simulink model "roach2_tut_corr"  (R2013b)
settings: Solver=VariableStepDiscrete  SolverMode=SingleTasking  StartTime=0.0  StopTime=100  RelTol=1e-3
undefined symbols (not defined in the file): add_latency, addr_width, Bit, bitfield, BitWidth, bram_latency, burst_size, casper_library_scopes, conv_latency, data_width, DelayLen, fan_latency, FFTSize, FFTStage, getfield, increment, led, Location, Lower, mult_latency, mux_latency, n_bits, n_bits_data, n_inputs, n_streams, n_taps, neg_latency, negate_latency, nsamples, pfb_size, pulse_len, reset_period, ROACH, ROACH2, snapshot, sx475t, sync_period, sync_period_bits, Upper, UseCounter, Width
libraries: xbsIndex_r4 x24444, casper_library_misc x73, xbsReplacements_r4 x34, casper_library_delays x14, xps_library x7
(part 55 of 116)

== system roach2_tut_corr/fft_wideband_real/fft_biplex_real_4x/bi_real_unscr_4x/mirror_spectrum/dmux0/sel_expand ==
  bus_in : Inport
  reinterpret{1..4} (4 alike) : xbsIndex_r4/Reinterpret  force_arith_type=on  arith_type=Unsigned  force_bin_pt=on  bin_pt=0  block_type=reinterpret
  slice1 : xbsIndex_r4/Slice  nbits=1  boolean_output=off  mode=Upper Bit Location + Width  bit1=-3  base1=MSB of Input  bit0=0  base0=LSB of Input  dbl_ovrd=off  block_type=slice
  slice2 : xbsIndex_r4/Slice  nbits=1  boolean_output=off  mode=Upper Bit Location + Width  bit1=-2  base1=MSB of Input  bit0=0  base0=LSB of Input  dbl_ovrd=off  block_type=slice
  slice3 : xbsIndex_r4/Slice  nbits=1  boolean_output=off  mode=Upper Bit Location + Width  bit1=-1  base1=MSB of Input  bit0=0  base0=LSB of Input  dbl_ovrd=off  block_type=slice
  slice4 : xbsIndex_r4/Slice  nbits=1  boolean_output=off  mode=Upper Bit Location + Width  bit1=0  base1=MSB of Input  bit0=0  base0=LSB of Input  dbl_ovrd=off  block_type=slice
  msb_out4 : Outport
  out3 : Outport  Port=2
  out2 : Outport  Port=3
  lsb_out1 : Outport  Port=4
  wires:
  bus_in/1 -> slice4/1, slice3/1, slice2/1, slice1/1
  slice4/1 -> reinterpret4/1
  reinterpret4/1 -> msb_out4/1
  slice3/1 -> reinterpret3/1
  reinterpret3/1 -> out3/1
  slice2/1 -> reinterpret2/1
  reinterpret2/1 -> out2/1
  slice1/1 -> reinterpret1/1
  reinterpret1/1 -> lsb_out1/1

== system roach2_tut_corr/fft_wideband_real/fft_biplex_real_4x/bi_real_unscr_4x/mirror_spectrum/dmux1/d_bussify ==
  in1 : Inport
  in2 : Inport  Port=2
  in3 : Inport  Port=3
  in4 : Inport  Port=4
  concatenate : xbsIndex_r4/Concat  num_inputs=4  dbl_ovrd=off  block_type=concat
  reinterpret{1..4} (4 alike) : xbsIndex_r4/Reinterpret  force_arith_type=on  arith_type=Unsigned  force_bin_pt=on  bin_pt=0  block_type=reinterpret
  bus_out : Outport
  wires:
  concatenate/1 -> bus_out/1
  in1/1 -> reinterpret1/1
  reinterpret1/1 -> concatenate/1
  in2/1 -> reinterpret2/1
  reinterpret2/1 -> concatenate/2
  in3/1 -> reinterpret3/1
  reinterpret3/1 -> concatenate/3
  in4/1 -> reinterpret4/1
  reinterpret4/1 -> concatenate/4

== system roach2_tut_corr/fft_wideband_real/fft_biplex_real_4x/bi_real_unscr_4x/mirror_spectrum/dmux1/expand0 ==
  bus_in : Inport
  reinterpret{1..4} (4 alike) : xbsIndex_r4/Reinterpret  force_arith_type=on  arith_type=Unsigned  force_bin_pt=on  bin_pt=0  block_type=reinterpret
  slice1 : xbsIndex_r4/Slice  nbits=36  boolean_output=off  mode=Upper Bit Location + Width  bit1=-108  base1=MSB of Input  bit0=0  base0=LSB of Input  dbl_ovrd=off  block_type=slice
  slice2 : xbsIndex_r4/Slice  nbits=36  boolean_output=off  mode=Upper Bit Location + Width  bit1=-72  base1=MSB of Input  bit0=0  base0=LSB of Input  dbl_ovrd=off  block_type=slice
  slice3 : xbsIndex_r4/Slice  nbits=36  boolean_output=off  mode=Upper Bit Location + Width  bit1=-36  base1=MSB of Input  bit0=0  base0=LSB of Input  dbl_ovrd=off  block_type=slice
  slice4 : xbsIndex_r4/Slice  nbits=36  boolean_output=off  mode=Upper Bit Location + Width  bit1=0  base1=MSB of Input  bit0=0  base0=LSB of Input  dbl_ovrd=off  block_type=slice
  msb_out4 : Outport
  out3 : Outport  Port=2
  out2 : Outport  Port=3
  lsb_out1 : Outport  Port=4
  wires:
  bus_in/1 -> slice4/1, slice3/1, slice2/1, slice1/1
  slice4/1 -> reinterpret4/1
  reinterpret4/1 -> msb_out4/1
  slice3/1 -> reinterpret3/1
  reinterpret3/1 -> out3/1
  slice2/1 -> reinterpret2/1
  reinterpret2/1 -> out2/1
  slice1/1 -> reinterpret1/1
  reinterpret1/1 -> lsb_out1/1

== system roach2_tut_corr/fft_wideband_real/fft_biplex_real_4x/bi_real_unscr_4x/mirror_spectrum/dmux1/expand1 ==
  bus_in : Inport
  reinterpret{1..4} (4 alike) : xbsIndex_r4/Reinterpret  force_arith_type=on  arith_type=Unsigned  force_bin_pt=on  bin_pt=0  block_type=reinterpret
  slice1 : xbsIndex_r4/Slice  nbits=36  boolean_output=off  mode=Upper Bit Location + Width  bit1=-108  base1=MSB of Input  bit0=0  base0=LSB of Input  dbl_ovrd=off  block_type=slice
  slice2 : xbsIndex_r4/Slice  nbits=36  boolean_output=off  mode=Upper Bit Location + Width  bit1=-72  base1=MSB of Input  bit0=0  base0=LSB of Input  dbl_ovrd=off  block_type=slice
  slice3 : xbsIndex_r4/Slice  nbits=36  boolean_output=off  mode=Upper Bit Location + Width  bit1=-36  base1=MSB of Input  bit0=0  base0=LSB of Input  dbl_ovrd=off  block_type=slice
  slice4 : xbsIndex_r4/Slice  nbits=36  boolean_output=off  mode=Upper Bit Location + Width  bit1=0  base1=MSB of Input  bit0=0  base0=LSB of Input  dbl_ovrd=off  block_type=slice
  msb_out4 : Outport
  out3 : Outport  Port=2
  out2 : Outport  Port=3
  lsb_out1 : Outport  Port=4
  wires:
  bus_in/1 -> slice4/1, slice3/1, slice2/1, slice1/1
  slice4/1 -> reinterpret4/1
  reinterpret4/1 -> msb_out4/1
  slice3/1 -> reinterpret3/1
  reinterpret3/1 -> out3/1
  slice2/1 -> reinterpret2/1
  reinterpret2/1 -> out2/1
  slice1/1 -> reinterpret1/1
  reinterpret1/1 -> lsb_out1/1

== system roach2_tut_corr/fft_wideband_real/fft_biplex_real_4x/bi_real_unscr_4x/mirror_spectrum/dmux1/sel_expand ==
  bus_in : Inport
  reinterpret{1..4} (4 alike) : xbsIndex_r4/Reinterpret  force_arith_type=on  arith_type=Unsigned  force_bin_pt=on  bin_pt=0  block_type=reinterpret
  slice1 : xbsIndex_r4/Slice  nbits=1  boolean_output=off  mode=Upper Bit Location + Width  bit1=-3  base1=MSB of Input  bit0=0  base0=LSB of Input  dbl_ovrd=off  block_type=slice
  slice2 : xbsIndex_r4/Slice  nbits=1  boolean_output=off  mode=Upper Bit Location + Width  bit1=-2  base1=MSB of Input  bit0=0  base0=LSB of Input  dbl_ovrd=off  block_type=slice
  slice3 : xbsIndex_r4/Slice  nbits=1  boolean_output=off  mode=Upper Bit Location + Width  bit1=-1  base1=MSB of Input  bit0=0  base0=LSB of Input  dbl_ovrd=off  block_type=slice
  slice4 : xbsIndex_r4/Slice  nbits=1  boolean_output=off  mode=Upper Bit Location + Width  bit1=0  base1=MSB of Input  bit0=0  base0=LSB of Input  dbl_ovrd=off  block_type=slice
  msb_out4 : Outport
  out3 : Outport  Port=2
  out2 : Outport  Port=3
  lsb_out1 : Outport  Port=4
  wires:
  bus_in/1 -> slice4/1, slice3/1, slice2/1, slice1/1
  slice4/1 -> reinterpret4/1
  reinterpret4/1 -> msb_out4/1
  slice3/1 -> reinterpret3/1
  reinterpret3/1 -> out3/1
  slice2/1 -> reinterpret2/1
  reinterpret2/1 -> out2/1
  slice1/1 -> reinterpret1/1
  reinterpret1/1 -> lsb_out1/1

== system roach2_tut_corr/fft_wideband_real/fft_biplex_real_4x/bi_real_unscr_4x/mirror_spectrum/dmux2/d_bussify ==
  in1 : Inport
  in2 : Inport  Port=2
  in3 : Inport  Port=3
  in4 : Inport  Port=4
  concatenate : xbsIndex_r4/Concat  num_inputs=4  dbl_ovrd=off  block_type=concat
  reinterpret{1..4} (4 alike) : xbsIndex_r4/Reinterpret  force_arith_type=on  arith_type=Unsigned  force_bin_pt=on  bin_pt=0  block_type=reinterpret
  bus_out : Outport
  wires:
  concatenate/1 -> bus_out/1
  in1/1 -> reinterpret1/1
  reinterpret1/1 -> concatenate/1
  in2/1 -> reinterpret2/1
  reinterpret2/1 -> concatenate/2
  in3/1 -> reinterpret3/1
  reinterpret3/1 -> concatenate/3
  in4/1 -> reinterpret4/1
  reinterpret4/1 -> concatenate/4

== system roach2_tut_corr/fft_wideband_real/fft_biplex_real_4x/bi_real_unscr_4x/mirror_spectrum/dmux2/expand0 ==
  bus_in : Inport
  reinterpret{1..4} (4 alike) : xbsIndex_r4/Reinterpret  force_arith_type=on  arith_type=Unsigned  force_bin_pt=on  bin_pt=0  block_type=reinterpret
  slice1 : xbsIndex_r4/Slice  nbits=36  boolean_output=off  mode=Upper Bit Location + Width  bit1=-108  base1=MSB of Input  bit0=0  base0=LSB of Input  dbl_ovrd=off  block_type=slice
  slice2 : xbsIndex_r4/Slice  nbits=36  boolean_output=off  mode=Upper Bit Location + Width  bit1=-72  base1=MSB of Input  bit0=0  base0=LSB of Input  dbl_ovrd=off  block_type=slice
  slice3 : xbsIndex_r4/Slice  nbits=36  boolean_output=off  mode=Upper Bit Location + Width  bit1=-36  base1=MSB of Input  bit0=0  base0=LSB of Input  dbl_ovrd=off  block_type=slice
  slice4 : xbsIndex_r4/Slice  nbits=36  boolean_output=off  mode=Upper Bit Location + Width  bit1=0  base1=MSB of Input  bit0=0  base0=LSB of Input  dbl_ovrd=off  block_type=slice
  msb_out4 : Outport
  out3 : Outport  Port=2
  out2 : Outport  Port=3
  lsb_out1 : Outport  Port=4
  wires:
  bus_in/1 -> slice4/1, slice3/1, slice2/1, slice1/1
  slice4/1 -> reinterpret4/1
  reinterpret4/1 -> msb_out4/1
  slice3/1 -> reinterpret3/1
  reinterpret3/1 -> out3/1
  slice2/1 -> reinterpret2/1
  reinterpret2/1 -> out2/1
  slice1/1 -> reinterpret1/1
  reinterpret1/1 -> lsb_out1/1

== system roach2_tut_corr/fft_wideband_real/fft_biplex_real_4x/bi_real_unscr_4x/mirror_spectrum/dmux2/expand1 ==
  bus_in : Inport
  reinterpret{1..4} (4 alike) : xbsIndex_r4/Reinterpret  force_arith_type=on  arith_type=Unsigned  force_bin_pt=on  bin_pt=0  block_type=reinterpret
  slice1 : xbsIndex_r4/Slice  nbits=36  boolean_output=off  mode=Upper Bit Location + Width  bit1=-108  base1=MSB of Input  bit0=0  base0=LSB of Input  dbl_ovrd=off  block_type=slice
  slice2 : xbsIndex_r4/Slice  nbits=36  boolean_output=off  mode=Upper Bit Location + Width  bit1=-72  base1=MSB of Input  bit0=0  base0=LSB of Input  dbl_ovrd=off  block_type=slice
  slice3 : xbsIndex_r4/Slice  nbits=36  boolean_output=off  mode=Upper Bit Location + Width  bit1=-36  base1=MSB of Input  bit0=0  base0=LSB of Input  dbl_ovrd=off  block_type=slice
  slice4 : xbsIndex_r4/Slice  nbits=36  boolean_output=off  mode=Upper Bit Location + Width  bit1=0  base1=MSB of Input  bit0=0  base0=LSB of Input  dbl_ovrd=off  block_type=slice
  msb_out4 : Outport
  out3 : Outport  Port=2
  out2 : Outport  Port=3
  lsb_out1 : Outport  Port=4
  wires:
  bus_in/1 -> slice4/1, slice3/1, slice2/1, slice1/1
  slice4/1 -> reinterpret4/1
  reinterpret4/1 -> msb_out4/1
  slice3/1 -> reinterpret3/1
  reinterpret3/1 -> out3/1
  slice2/1 -> reinterpret2/1
  reinterpret2/1 -> out2/1
  slice1/1 -> reinterpret1/1
  reinterpret1/1 -> lsb_out1/1

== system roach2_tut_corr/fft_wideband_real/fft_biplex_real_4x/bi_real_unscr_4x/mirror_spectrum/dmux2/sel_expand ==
  bus_in : Inport
  reinterpret{1..4} (4 alike) : xbsIndex_r4/Reinterpret  force_arith_type=on  arith_type=Unsigned  force_bin_pt=on  bin_pt=0  block_type=reinterpret
  slice1 : xbsIndex_r4/Slice  nbits=1  boolean_output=off  mode=Upper Bit Location + Width  bit1=-3  base1=MSB of Input  bit0=0  base0=LSB of Input  dbl_ovrd=off  block_type=slice
  slice2 : xbsIndex_r4/Slice  nbits=1  boolean_output=off  mode=Upper Bit Location + Width  bit1=-2  base1=MSB of Input  bit0=0  base0=LSB of Input  dbl_ovrd=off  block_type=slice
  slice3 : xbsIndex_r4/Slice  nbits=1  boolean_output=off  mode=Upper Bit Location + Width  bit1=-1  base1=MSB of Input  bit0=0  base0=LSB of Input  dbl_ovrd=off  block_type=slice
  slice4 : xbsIndex_r4/Slice  nbits=1  boolean_output=off  mode=Upper Bit Location + Width  bit1=0  base1=MSB of Input  bit0=0  base0=LSB of Input  dbl_ovrd=off  block_type=slice
  msb_out4 : Outport
  out3 : Outport  Port=2
  out2 : Outport  Port=3
  lsb_out1 : Outport  Port=4
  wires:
  bus_in/1 -> slice4/1, slice3/1, slice2/1, slice1/1
  slice4/1 -> reinterpret4/1
  reinterpret4/1 -> msb_out4/1
  slice3/1 -> reinterpret3/1
  reinterpret3/1 -> out3/1
  slice2/1 -> reinterpret2/1
  reinterpret2/1 -> out2/1
  slice1/1 -> reinterpret1/1
  reinterpret1/1 -> lsb_out1/1

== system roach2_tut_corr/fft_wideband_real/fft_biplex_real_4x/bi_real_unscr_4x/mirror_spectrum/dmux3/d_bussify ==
  in1 : Inport
  in2 : Inport  Port=2
  in3 : Inport  Port=3
  in4 : Inport  Port=4
  concatenate : xbsIndex_r4/Concat  num_inputs=4  dbl_ovrd=off  block_type=concat
  reinterpret{1..4} (4 alike) : xbsIndex_r4/Reinterpret  force_arith_type=on  arith_type=Unsigned  force_bin_pt=on  bin_pt=0  block_type=reinterpret
  bus_out : Outport
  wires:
  concatenate/1 -> bus_out/1
  in1/1 -> reinterpret1/1
  reinterpret1/1 -> concatenate/1
  in2/1 -> reinterpret2/1
  reinterpret2/1 -> concatenate/2
  in3/1 -> reinterpret3/1
  reinterpret3/1 -> concatenate/3
  in4/1 -> reinterpret4/1
  reinterpret4/1 -> concatenate/4

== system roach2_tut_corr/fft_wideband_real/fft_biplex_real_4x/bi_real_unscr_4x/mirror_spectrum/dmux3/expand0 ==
  bus_in : Inport
  reinterpret{1..4} (4 alike) : xbsIndex_r4/Reinterpret  force_arith_type=on  arith_type=Unsigned  force_bin_pt=on  bin_pt=0  block_type=reinterpret
  slice1 : xbsIndex_r4/Slice  nbits=36  boolean_output=off  mode=Upper Bit Location + Width  bit1=-108  base1=MSB of Input  bit0=0  base0=LSB of Input  dbl_ovrd=off  block_type=slice
  slice2 : xbsIndex_r4/Slice  nbits=36  boolean_output=off  mode=Upper Bit Location + Width  bit1=-72  base1=MSB of Input  bit0=0  base0=LSB of Input  dbl_ovrd=off  block_type=slice
  slice3 : xbsIndex_r4/Slice  nbits=36  boolean_output=off  mode=Upper Bit Location + Width  bit1=-36  base1=MSB of Input  bit0=0  base0=LSB of Input  dbl_ovrd=off  block_type=slice
  slice4 : xbsIndex_r4/Slice  nbits=36  boolean_output=off  mode=Upper Bit Location + Width  bit1=0  base1=MSB of Input  bit0=0  base0=LSB of Input  dbl_ovrd=off  block_type=slice
  msb_out4 : Outport
  out3 : Outport  Port=2
  out2 : Outport  Port=3
  lsb_out1 : Outport  Port=4
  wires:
  bus_in/1 -> slice4/1, slice3/1, slice2/1, slice1/1
  slice4/1 -> reinterpret4/1
  reinterpret4/1 -> msb_out4/1
  slice3/1 -> reinterpret3/1
  reinterpret3/1 -> out3/1
  slice2/1 -> reinterpret2/1
  reinterpret2/1 -> out2/1
  slice1/1 -> reinterpret1/1
  reinterpret1/1 -> lsb_out1/1

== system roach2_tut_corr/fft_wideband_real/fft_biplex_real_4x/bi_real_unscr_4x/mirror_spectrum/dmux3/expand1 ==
  bus_in : Inport
  reinterpret{1..4} (4 alike) : xbsIndex_r4/Reinterpret  force_arith_type=on  arith_type=Unsigned  force_bin_pt=on  bin_pt=0  block_type=reinterpret
  slice1 : xbsIndex_r4/Slice  nbits=36  boolean_output=off  mode=Upper Bit Location + Width  bit1=-108  base1=MSB of Input  bit0=0  base0=LSB of Input  dbl_ovrd=off  block_type=slice
  slice2 : xbsIndex_r4/Slice  nbits=36  boolean_output=off  mode=Upper Bit Location + Width  bit1=-72  base1=MSB of Input  bit0=0  base0=LSB of Input  dbl_ovrd=off  block_type=slice
  slice3 : xbsIndex_r4/Slice  nbits=36  boolean_output=off  mode=Upper Bit Location + Width  bit1=-36  base1=MSB of Input  bit0=0  base0=LSB of Input  dbl_ovrd=off  block_type=slice
  slice4 : xbsIndex_r4/Slice  nbits=36  boolean_output=off  mode=Upper Bit Location + Width  bit1=0  base1=MSB of Input  bit0=0  base0=LSB of Input  dbl_ovrd=off  block_type=slice
  msb_out4 : Outport
  out3 : Outport  Port=2
  out2 : Outport  Port=3
  lsb_out1 : Outport  Port=4
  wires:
  bus_in/1 -> slice4/1, slice3/1, slice2/1, slice1/1
  slice4/1 -> reinterpret4/1
  reinterpret4/1 -> msb_out4/1
  slice3/1 -> reinterpret3/1
  reinterpret3/1 -> out3/1
  slice2/1 -> reinterpret2/1
  reinterpret2/1 -> out2/1
  slice1/1 -> reinterpret1/1
  reinterpret1/1 -> lsb_out1/1

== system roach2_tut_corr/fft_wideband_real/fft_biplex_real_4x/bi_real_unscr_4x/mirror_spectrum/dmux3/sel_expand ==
  bus_in : Inport
  reinterpret{1..4} (4 alike) : xbsIndex_r4/Reinterpret  force_arith_type=on  arith_type=Unsigned  force_bin_pt=on  bin_pt=0  block_type=reinterpret
  slice1 : xbsIndex_r4/Slice  nbits=1  boolean_output=off  mode=Upper Bit Location + Width  bit1=-3  base1=MSB of Input  bit0=0  base0=LSB of Input  dbl_ovrd=off  block_type=slice
  slice2 : xbsIndex_r4/Slice  nbits=1  boolean_output=off  mode=Upper Bit Location + Width  bit1=-2  base1=MSB of Input  bit0=0  base0=LSB of Input  dbl_ovrd=off  block_type=slice
  slice3 : xbsIndex_r4/Slice  nbits=1  boolean_output=off  mode=Upper Bit Location + Width  bit1=-1  base1=MSB of Input  bit0=0  base0=LSB of Input  dbl_ovrd=off  block_type=slice
  slice4 : xbsIndex_r4/Slice  nbits=1  boolean_output=off  mode=Upper Bit Location + Width  bit1=0  base1=MSB of Input  bit0=0  base0=LSB of Input  dbl_ovrd=off  block_type=slice
  msb_out4 : Outport
  out3 : Outport  Port=2
  out2 : Outport  Port=3
  lsb_out1 : Outport  Port=4
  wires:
  bus_in/1 -> slice4/1, slice3/1, slice2/1, slice1/1
  slice4/1 -> reinterpret4/1
  reinterpret4/1 -> msb_out4/1
  slice3/1 -> reinterpret3/1
  reinterpret3/1 -> out3/1
  slice2/1 -> reinterpret2/1
  reinterpret2/1 -> out2/1
  slice1/1 -> reinterpret1/1
  reinterpret1/1 -> lsb_out1/1

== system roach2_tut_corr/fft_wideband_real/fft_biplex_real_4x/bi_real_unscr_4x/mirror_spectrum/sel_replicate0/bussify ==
  in1 : Inport
  in2 : Inport  Port=2
  in3 : Inport  Port=3
  in4 : Inport  Port=4
  concatenate : xbsIndex_r4/Concat  num_inputs=4  dbl_ovrd=off  block_type=concat
  reinterpret{1..4} (4 alike) : xbsIndex_r4/Reinterpret  force_arith_type=on  arith_type=Unsigned  force_bin_pt=on  bin_pt=0  block_type=reinterpret
  bus_out : Outport
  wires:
  concatenate/1 -> bus_out/1
  in1/1 -> reinterpret1/1
  reinterpret1/1 -> concatenate/1
  in2/1 -> reinterpret2/1
  reinterpret2/1 -> concatenate/2
  in3/1 -> reinterpret3/1
  reinterpret3/1 -> concatenate/3
  in4/1 -> reinterpret4/1
  reinterpret4/1 -> concatenate/4

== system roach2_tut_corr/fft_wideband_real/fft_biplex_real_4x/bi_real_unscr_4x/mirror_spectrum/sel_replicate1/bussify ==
  in1 : Inport
  in2 : Inport  Port=2
  in3 : Inport  Port=3
  in4 : Inport  Port=4
  concatenate : xbsIndex_r4/Concat  num_inputs=4  dbl_ovrd=off  block_type=concat
  reinterpret{1..4} (4 alike) : xbsIndex_r4/Reinterpret  force_arith_type=on  arith_type=Unsigned  force_bin_pt=on  bin_pt=0  block_type=reinterpret
  bus_out : Outport
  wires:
  concatenate/1 -> bus_out/1
  in1/1 -> reinterpret1/1
  reinterpret1/1 -> concatenate/1
  in2/1 -> reinterpret2/1
  reinterpret2/1 -> concatenate/2
  in3/1 -> reinterpret3/1
  reinterpret3/1 -> concatenate/3
  in4/1 -> reinterpret4/1
  reinterpret4/1 -> concatenate/4

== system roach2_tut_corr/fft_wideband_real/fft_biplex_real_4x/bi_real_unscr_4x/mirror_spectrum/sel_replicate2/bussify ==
  in1 : Inport
  in2 : Inport  Port=2
  in3 : Inport  Port=3
  in4 : Inport  Port=4
  concatenate : xbsIndex_r4/Concat  num_inputs=4  dbl_ovrd=off  block_type=concat
  reinterpret{1..4} (4 alike) : xbsIndex_r4/Reinterpret  force_arith_type=on  arith_type=Unsigned  force_bin_pt=on  bin_pt=0  block_type=reinterpret
  bus_out : Outport
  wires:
  concatenate/1 -> bus_out/1
  in1/1 -> reinterpret1/1
  reinterpret1/1 -> concatenate/1
  in2/1 -> reinterpret2/1
  reinterpret2/1 -> concatenate/2
  in3/1 -> reinterpret3/1
  reinterpret3/1 -> concatenate/3
  in4/1 -> reinterpret4/1
  reinterpret4/1 -> concatenate/4

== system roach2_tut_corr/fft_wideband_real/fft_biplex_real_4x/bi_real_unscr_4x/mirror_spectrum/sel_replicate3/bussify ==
  in1 : Inport
  in2 : Inport  Port=2
  in3 : Inport  Port=3
  in4 : Inport  Port=4
  concatenate : xbsIndex_r4/Concat  num_inputs=4  dbl_ovrd=off  block_type=concat
  reinterpret{1..4} (4 alike) : xbsIndex_r4/Reinterpret  force_arith_type=on  arith_type=Unsigned  force_bin_pt=on  bin_pt=0  block_type=reinterpret
  bus_out : Outport
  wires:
  concatenate/1 -> bus_out/1
  in1/1 -> reinterpret1/1
  reinterpret1/1 -> concatenate/1
  in2/1 -> reinterpret2/1
  reinterpret2/1 -> concatenate/2
  in3/1 -> reinterpret3/1
  reinterpret3/1 -> concatenate/3
  in4/1 -> reinterpret4/1
  reinterpret4/1 -> concatenate/4

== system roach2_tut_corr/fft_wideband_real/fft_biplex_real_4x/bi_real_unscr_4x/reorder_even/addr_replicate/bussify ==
  in1 : Inport
  reinterpret1 : xbsIndex_r4/Reinterpret  force_arith_type=on  arith_type=Unsigned  force_bin_pt=on  bin_pt=0  block_type=reinterpret
  bus_out : Outport
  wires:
  in1/1 -> reinterpret1/1
  reinterpret1/1 -> bus_out/1

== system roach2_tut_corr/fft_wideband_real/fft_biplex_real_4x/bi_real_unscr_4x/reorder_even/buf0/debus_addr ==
  bus_in : Inport
  reinterpret{1..4} (4 alike) : xbsIndex_r4/Reinterpret  force_arith_type=on  arith_type=Unsigned  force_bin_pt=on  bin_pt=0  block_type=reinterpret
  slice1 : xbsIndex_r4/Slice  nbits=8  boolean_output=off  mode=Upper Bit Location + Width  bit1=-24  base1=MSB of Input  bit0=0  base0=LSB of Input  dbl_ovrd=off  block_type=slice
  slice2 : xbsIndex_r4/Slice  nbits=8  boolean_output=off  mode=Upper Bit Location + Width  bit1=-16  base1=MSB of Input  bit0=0  base0=LSB of Input  dbl_ovrd=off  block_type=slice
  slice3 : xbsIndex_r4/Slice  nbits=8  boolean_output=off  mode=Upper Bit Location + Width  bit1=-8  base1=MSB of Input  bit0=0  base0=LSB of Input  dbl_ovrd=off  block_type=slice
  slice4 : xbsIndex_r4/Slice  nbits=8  boolean_output=off  mode=Upper Bit Location + Width  bit1=0  base1=MSB of Input  bit0=0  base0=LSB of Input  dbl_ovrd=off  block_type=slice
  msb_out4 : Outport
  out3 : Outport  Port=2
  out2 : Outport  Port=3
  lsb_out1 : Outport  Port=4
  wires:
  bus_in/1 -> slice4/1, slice3/1, slice2/1, slice1/1
  slice4/1 -> reinterpret4/1
  reinterpret4/1 -> msb_out4/1
  slice3/1 -> reinterpret3/1
  reinterpret3/1 -> out3/1
  slice2/1 -> reinterpret2/1
  reinterpret2/1 -> out2/1
  slice1/1 -> reinterpret1/1
  reinterpret1/1 -> lsb_out1/1

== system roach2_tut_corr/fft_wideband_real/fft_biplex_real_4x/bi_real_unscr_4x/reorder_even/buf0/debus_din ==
  bus_in : Inport
  reinterpret{1..4} (4 alike) : xbsIndex_r4/Reinterpret  force_arith_type=on  arith_type=Unsigned  force_bin_pt=on  bin_pt=0  block_type=reinterpret
  slice1 : xbsIndex_r4/Slice  nbits=36  boolean_output=off  mode=Upper Bit Location + Width  bit1=-108  base1=MSB of Input  bit0=0  base0=LSB of Input  dbl_ovrd=off  block_type=slice
  slice2 : xbsIndex_r4/Slice  nbits=36  boolean_output=off  mode=Upper Bit Location + Width  bit1=-72  base1=MSB of Input  bit0=0  base0=LSB of Input  dbl_ovrd=off  block_type=slice
  slice3 : xbsIndex_r4/Slice  nbits=36  boolean_output=off  mode=Upper Bit Location + Width  bit1=-36  base1=MSB of Input  bit0=0  base0=LSB of Input  dbl_ovrd=off  block_type=slice
  slice4 : xbsIndex_r4/Slice  nbits=36  boolean_output=off  mode=Upper Bit Location + Width  bit1=0  base1=MSB of Input  bit0=0  base0=LSB of Input  dbl_ovrd=off  block_type=slice
  msb_out4 : Outport
  out3 : Outport  Port=2
  out2 : Outport  Port=3
  lsb_out1 : Outport  Port=4
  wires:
  bus_in/1 -> slice4/1, slice3/1, slice2/1, slice1/1
  slice4/1 -> reinterpret4/1
  reinterpret4/1 -> msb_out4/1
  slice3/1 -> reinterpret3/1
  reinterpret3/1 -> out3/1
  slice2/1 -> reinterpret2/1
  reinterpret2/1 -> out2/1
  slice1/1 -> reinterpret1/1
  reinterpret1/1 -> lsb_out1/1

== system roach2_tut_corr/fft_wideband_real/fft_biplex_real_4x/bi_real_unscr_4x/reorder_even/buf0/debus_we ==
  bus_in : Inport
  slice1 : xbsIndex_r4/Slice  nbits=1  boolean_output=on  mode=Upper Bit Location + Width  bit1=-3  base1=MSB of Input  bit0=0  base0=LSB of Input  dbl_ovrd=off  block_type=slice
  slice2 : xbsIndex_r4/Slice  nbits=1  boolean_output=on  mode=Upper Bit Location + Width  bit1=-2  base1=MSB of Input  bit0=0  base0=LSB of Input  dbl_ovrd=off  block_type=slice
  slice3 : xbsIndex_r4/Slice  nbits=1  boolean_output=on  mode=Upper Bit Location + Width  bit1=-1  base1=MSB of Input  bit0=0  base0=LSB of Input  dbl_ovrd=off  block_type=slice
  slice4 : xbsIndex_r4/Slice  nbits=1  boolean_output=on  mode=Upper Bit Location + Width  bit1=0  base1=MSB of Input  bit0=0  base0=LSB of Input  dbl_ovrd=off  block_type=slice
  msb_out4 : Outport
  out3 : Outport  Port=2
  out2 : Outport  Port=3
  lsb_out1 : Outport  Port=4
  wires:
  bus_in/1 -> slice4/1, slice3/1, slice2/1, slice1/1
  slice4/1 -> msb_out4/1
  slice3/1 -> out3/1
  slice2/1 -> out2/1
  slice1/1 -> lsb_out1/1

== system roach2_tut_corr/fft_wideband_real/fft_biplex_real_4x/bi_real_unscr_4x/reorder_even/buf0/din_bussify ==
  in1 : Inport
  in2 : Inport  Port=2
  in3 : Inport  Port=3
  in4 : Inport  Port=4
  concatenate : xbsIndex_r4/Concat  num_inputs=4  dbl_ovrd=off  block_type=concat
  reinterpret{1..4} (4 alike) : xbsIndex_r4/Reinterpret  force_arith_type=on  arith_type=Unsigned  force_bin_pt=on  bin_pt=0  block_type=reinterpret
  bus_out : Outport
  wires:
  concatenate/1 -> bus_out/1
  in1/1 -> reinterpret1/1
  reinterpret1/1 -> concatenate/1
  in2/1 -> reinterpret2/1
  reinterpret2/1 -> concatenate/2
  in3/1 -> reinterpret3/1
  reinterpret3/1 -> concatenate/3
  in4/1 -> reinterpret4/1
  reinterpret4/1 -> concatenate/4

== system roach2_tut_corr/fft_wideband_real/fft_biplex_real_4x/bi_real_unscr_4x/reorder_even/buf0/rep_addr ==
  in : Inport
  bussify : Subsystem  AncestorBlock=casper_library_flow_control/bus_create
  din0_0 : xbsIndex_r4/Delay  rst=off  infoeditControl=Selection of Reset will increase slice count due to use of real FFs and instead of SRLs  en=off  latency=1  dbl_ovrd=off  reg_retiming=off  block_type=delay
  din0_1 : xbsIndex_r4/Delay  rst=off  infoeditControl=Selection of Reset will increase slice count due to use of real FFs and instead of SRLs  en=off  latency=1  dbl_ovrd=off  reg_retiming=off  block_type=delay
  din1_{0..3} (4 alike) : xbsIndex_r4/Delay  rst=off  infoeditControl=Selection of Reset will increase slice count due to use of real FFs and instead of SRLs  en=off  latency=1  dbl_ovrd=off  reg_retiming=off  block_type=delay
  out : Outport
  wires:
  in/1 -> din0_0/1, din0_1/1
  din0_0/1 -> din1_0/1, din1_2/1
  din0_1/1 -> din1_1/1, din1_3/1
  din1_0/1 -> bussify/1(in1)
  din1_1/1 -> bussify/2(in2)
  din1_2/1 -> bussify/3(in3)
  din1_3/1 -> bussify/4(in4)
  bussify/1(bus_out) -> out/1

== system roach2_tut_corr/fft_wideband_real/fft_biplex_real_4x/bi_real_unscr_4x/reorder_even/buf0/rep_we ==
  in : Inport
  bussify : Subsystem  AncestorBlock=casper_library_flow_control/bus_create
  din0_0 : xbsIndex_r4/Delay  rst=off  infoeditControl=Selection of Reset will increase slice count due to use of real FFs and instead of SRLs  en=off  latency=1  dbl_ovrd=off  reg_retiming=off  block_type=delay
  din0_1 : xbsIndex_r4/Delay  rst=off  infoeditControl=Selection of Reset will increase slice count due to use of real FFs and instead of SRLs  en=off  latency=1  dbl_ovrd=off  reg_retiming=off  block_type=delay
  din1_{0..3} (4 alike) : xbsIndex_r4/Delay  rst=off  infoeditControl=Selection of Reset will increase slice count due to use of real FFs and instead of SRLs  en=off  latency=1  dbl_ovrd=off  reg_retiming=off  block_type=delay
  out : Outport
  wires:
  in/1 -> din0_0/1, din0_1/1
  din0_0/1 -> din1_0/1, din1_2/1
  din0_1/1 -> din1_1/1, din1_3/1
  din1_0/1 -> bussify/1(in1)
  din1_1/1 -> bussify/2(in2)
  din1_2/1 -> bussify/3(in3)
  din1_3/1 -> bussify/4(in4)
  bussify/1(bus_out) -> out/1

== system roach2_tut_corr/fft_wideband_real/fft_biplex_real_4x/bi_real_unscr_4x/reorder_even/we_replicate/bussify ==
  in1 : Inport
  reinterpret1 : xbsIndex_r4/Reinterpret  force_arith_type=on  arith_type=Unsigned  force_bin_pt=on  bin_pt=0  block_type=reinterpret
  bus_out : Outport
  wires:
  in1/1 -> reinterpret1/1
  reinterpret1/1 -> bus_out/1

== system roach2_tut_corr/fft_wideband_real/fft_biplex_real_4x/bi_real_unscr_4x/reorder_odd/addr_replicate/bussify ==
  in1 : Inport
  reinterpret1 : xbsIndex_r4/Reinterpret  force_arith_type=on  arith_type=Unsigned  force_bin_pt=on  bin_pt=0  block_type=reinterpret
  bus_out : Outport
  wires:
  in1/1 -> reinterpret1/1
  reinterpret1/1 -> bus_out/1

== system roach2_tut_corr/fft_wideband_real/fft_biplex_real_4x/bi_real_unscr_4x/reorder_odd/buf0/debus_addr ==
  bus_in : Inport
  reinterpret{1..4} (4 alike) : xbsIndex_r4/Reinterpret  force_arith_type=on  arith_type=Unsigned  force_bin_pt=on  bin_pt=0  block_type=reinterpret
  slice1 : xbsIndex_r4/Slice  nbits=8  boolean_output=off  mode=Upper Bit Location + Width  bit1=-24  base1=MSB of Input  bit0=0  base0=LSB of Input  dbl_ovrd=off  block_type=slice
  slice2 : xbsIndex_r4/Slice  nbits=8  boolean_output=off  mode=Upper Bit Location + Width  bit1=-16  base1=MSB of Input  bit0=0  base0=LSB of Input  dbl_ovrd=off  block_type=slice
  slice3 : xbsIndex_r4/Slice  nbits=8  boolean_output=off  mode=Upper Bit Location + Width  bit1=-8  base1=MSB of Input  bit0=0  base0=LSB of Input  dbl_ovrd=off  block_type=slice
  slice4 : xbsIndex_r4/Slice  nbits=8  boolean_output=off  mode=Upper Bit Location + Width  bit1=0  base1=MSB of Input  bit0=0  base0=LSB of Input  dbl_ovrd=off  block_type=slice
  msb_out4 : Outport
  out3 : Outport  Port=2
  out2 : Outport  Port=3
  lsb_out1 : Outport  Port=4
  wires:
  bus_in/1 -> slice4/1, slice3/1, slice2/1, slice1/1
  slice4/1 -> reinterpret4/1
  reinterpret4/1 -> msb_out4/1
  slice3/1 -> reinterpret3/1
  reinterpret3/1 -> out3/1
  slice2/1 -> reinterpret2/1
  reinterpret2/1 -> out2/1
  slice1/1 -> reinterpret1/1
  reinterpret1/1 -> lsb_out1/1

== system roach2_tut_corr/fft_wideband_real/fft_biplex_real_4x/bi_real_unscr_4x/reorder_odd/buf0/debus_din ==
  bus_in : Inport
  reinterpret{1..4} (4 alike) : xbsIndex_r4/Reinterpret  force_arith_type=on  arith_type=Unsigned  force_bin_pt=on  bin_pt=0  block_type=reinterpret
  slice1 : xbsIndex_r4/Slice  nbits=36  boolean_output=off  mode=Upper Bit Location + Width  bit1=-108  base1=MSB of Input  bit0=0  base0=LSB of Input  dbl_ovrd=off  block_type=slice
  slice2 : xbsIndex_r4/Slice  nbits=36  boolean_output=off  mode=Upper Bit Location + Width  bit1=-72  base1=MSB of Input  bit0=0  base0=LSB of Input  dbl_ovrd=off  block_type=slice
  slice3 : xbsIndex_r4/Slice  nbits=36  boolean_output=off  mode=Upper Bit Location + Width  bit1=-36  base1=MSB of Input  bit0=0  base0=LSB of Input  dbl_ovrd=off  block_type=slice
  slice4 : xbsIndex_r4/Slice  nbits=36  boolean_output=off  mode=Upper Bit Location + Width  bit1=0  base1=MSB of Input  bit0=0  base0=LSB of Input  dbl_ovrd=off  block_type=slice
  msb_out4 : Outport
  out3 : Outport  Port=2
  out2 : Outport  Port=3
  lsb_out1 : Outport  Port=4
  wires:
  bus_in/1 -> slice4/1, slice3/1, slice2/1, slice1/1
  slice4/1 -> reinterpret4/1
  reinterpret4/1 -> msb_out4/1
  slice3/1 -> reinterpret3/1
  reinterpret3/1 -> out3/1
  slice2/1 -> reinterpret2/1
  reinterpret2/1 -> out2/1
  slice1/1 -> reinterpret1/1
  reinterpret1/1 -> lsb_out1/1

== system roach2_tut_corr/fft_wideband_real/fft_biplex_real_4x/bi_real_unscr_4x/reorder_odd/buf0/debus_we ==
  bus_in : Inport
  slice1 : xbsIndex_r4/Slice  nbits=1  boolean_output=on  mode=Upper Bit Location + Width  bit1=-3  base1=MSB of Input  bit0=0  base0=LSB of Input  dbl_ovrd=off  block_type=slice
  slice2 : xbsIndex_r4/Slice  nbits=1  boolean_output=on  mode=Upper Bit Location + Width  bit1=-2  base1=MSB of Input  bit0=0  base0=LSB of Input  dbl_ovrd=off  block_type=slice
  slice3 : xbsIndex_r4/Slice  nbits=1  boolean_output=on  mode=Upper Bit Location + Width  bit1=-1  base1=MSB of Input  bit0=0  base0=LSB of Input  dbl_ovrd=off  block_type=slice
  slice4 : xbsIndex_r4/Slice  nbits=1  boolean_output=on  mode=Upper Bit Location + Width  bit1=0  base1=MSB of Input  bit0=0  base0=LSB of Input  dbl_ovrd=off  block_type=slice
  msb_out4 : Outport
  out3 : Outport  Port=2
  out2 : Outport  Port=3
  lsb_out1 : Outport  Port=4
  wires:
  bus_in/1 -> slice4/1, slice3/1, slice2/1, slice1/1
  slice4/1 -> msb_out4/1
  slice3/1 -> out3/1
  slice2/1 -> out2/1
  slice1/1 -> lsb_out1/1

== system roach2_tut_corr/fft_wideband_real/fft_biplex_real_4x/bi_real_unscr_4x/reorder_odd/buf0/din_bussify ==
  in1 : Inport
  in2 : Inport  Port=2
  in3 : Inport  Port=3
  in4 : Inport  Port=4
  concatenate : xbsIndex_r4/Concat  num_inputs=4  dbl_ovrd=off  block_type=concat
  reinterpret{1..4} (4 alike) : xbsIndex_r4/Reinterpret  force_arith_type=on  arith_type=Unsigned  force_bin_pt=on  bin_pt=0  block_type=reinterpret
  bus_out : Outport
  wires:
  concatenate/1 -> bus_out/1
  in1/1 -> reinterpret1/1
  reinterpret1/1 -> concatenate/1
  in2/1 -> reinterpret2/1
  reinterpret2/1 -> concatenate/2
  in3/1 -> reinterpret3/1
  reinterpret3/1 -> concatenate/3
  in4/1 -> reinterpret4/1
  reinterpret4/1 -> concatenate/4

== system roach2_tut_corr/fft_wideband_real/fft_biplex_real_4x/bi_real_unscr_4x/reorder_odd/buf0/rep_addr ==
  in : Inport
  bussify : Subsystem  AncestorBlock=casper_library_flow_control/bus_create
  din0_0 : xbsIndex_r4/Delay  rst=off  infoeditControl=Selection of Reset will increase slice count due to use of real FFs and instead of SRLs  en=off  latency=1  dbl_ovrd=off  reg_retiming=off  block_type=delay
  din0_1 : xbsIndex_r4/Delay  rst=off  infoeditControl=Selection of Reset will increase slice count due to use of real FFs and instead of SRLs  en=off  latency=1  dbl_ovrd=off  reg_retiming=off  block_type=delay
  din1_{0..3} (4 alike) : xbsIndex_r4/Delay  rst=off  infoeditControl=Selection of Reset will increase slice count due to use of real FFs and instead of SRLs  en=off  latency=1  dbl_ovrd=off  reg_retiming=off  block_type=delay
  out : Outport
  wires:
  in/1 -> din0_0/1, din0_1/1
  din0_0/1 -> din1_0/1, din1_2/1
  din0_1/1 -> din1_1/1, din1_3/1
  din1_0/1 -> bussify/1(in1)
  din1_1/1 -> bussify/2(in2)
  din1_2/1 -> bussify/3(in3)
  din1_3/1 -> bussify/4(in4)
  bussify/1(bus_out) -> out/1

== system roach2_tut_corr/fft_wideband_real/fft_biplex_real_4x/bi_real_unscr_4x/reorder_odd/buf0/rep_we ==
  in : Inport
  bussify : Subsystem  AncestorBlock=casper_library_flow_control/bus_create
  din0_0 : xbsIndex_r4/Delay  rst=off  infoeditControl=Selection of Reset will increase slice count due to use of real FFs and instead of SRLs  en=off  latency=1  dbl_ovrd=off  reg_retiming=off  block_type=delay
  din0_1 : xbsIndex_r4/Delay  rst=off  infoeditControl=Selection of Reset will increase slice count due to use of real FFs and instead of SRLs  en=off  latency=1  dbl_ovrd=off  reg_retiming=off  block_type=delay
  din1_{0..3} (4 alike) : xbsIndex_r4/Delay  rst=off  infoeditControl=Selection of Reset will increase slice count due to use of real FFs and instead of SRLs  en=off  latency=1  dbl_ovrd=off  reg_retiming=off  block_type=delay
  out : Outport
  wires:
  in/1 -> din0_0/1, din0_1/1
  din0_0/1 -> din1_0/1, din1_2/1
  din0_1/1 -> din1_1/1, din1_3/1
  din1_0/1 -> bussify/1(in1)
  din1_1/1 -> bussify/2(in2)
  din1_2/1 -> bussify/3(in3)
  din1_3/1 -> bussify/4(in4)
  bussify/1(bus_out) -> out/1

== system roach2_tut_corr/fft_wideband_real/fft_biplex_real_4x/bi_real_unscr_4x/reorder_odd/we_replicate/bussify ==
  in1 : Inport
  reinterpret1 : xbsIndex_r4/Reinterpret  force_arith_type=on  arith_type=Unsigned  force_bin_pt=on  bin_pt=0  block_type=reinterpret
  bus_out : Outport
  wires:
  in1/1 -> reinterpret1/1
  reinterpret1/1 -> bus_out/1

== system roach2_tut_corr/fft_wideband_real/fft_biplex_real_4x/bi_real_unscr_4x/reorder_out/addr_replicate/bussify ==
  in1 : Inport
  in2 : Inport  Port=2
  in3 : Inport  Port=3
  in4 : Inport  Port=4
  concatenate : xbsIndex_r4/Concat  num_inputs=4  dbl_ovrd=off  block_type=concat
  reinterpret{1..4} (4 alike) : xbsIndex_r4/Reinterpret  force_arith_type=on  arith_type=Unsigned  force_bin_pt=on  bin_pt=0  block_type=reinterpret
  bus_out : Outport
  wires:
  concatenate/1 -> bus_out/1
  in1/1 -> reinterpret1/1
  reinterpret1/1 -> concatenate/1
  in2/1 -> reinterpret2/1
  reinterpret2/1 -> concatenate/2
  in3/1 -> reinterpret3/1
  reinterpret3/1 -> concatenate/3
  in4/1 -> reinterpret4/1
  reinterpret4/1 -> concatenate/4

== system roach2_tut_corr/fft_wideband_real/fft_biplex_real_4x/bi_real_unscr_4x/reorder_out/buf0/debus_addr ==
  bus_in : Inport
  reinterpret{1..4} (4 alike) : xbsIndex_r4/Reinterpret  force_arith_type=on  arith_type=Unsigned  force_bin_pt=on  bin_pt=0  block_type=reinterpret
  slice1 : xbsIndex_r4/Slice  nbits=8  boolean_output=off  mode=Upper Bit Location + Width  bit1=-24  base1=MSB of Input  bit0=0  base0=LSB of Input  dbl_ovrd=off  block_type=slice
  slice2 : xbsIndex_r4/Slice  nbits=8  boolean_output=off  mode=Upper Bit Location + Width  bit1=-16  base1=MSB of Input  bit0=0  base0=LSB of Input  dbl_ovrd=off  block_type=slice
  slice3 : xbsIndex_r4/Slice  nbits=8  boolean_output=off  mode=Upper Bit Location + Width  bit1=-8  base1=MSB of Input  bit0=0  base0=LSB of Input  dbl_ovrd=off  block_type=slice
  slice4 : xbsIndex_r4/Slice  nbits=8  boolean_output=off  mode=Upper Bit Location + Width  bit1=0  base1=MSB of Input  bit0=0  base0=LSB of Input  dbl_ovrd=off  block_type=slice
  msb_out4 : Outport
  out3 : Outport  Port=2
  out2 : Outport  Port=3
  lsb_out1 : Outport  Port=4
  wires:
  bus_in/1 -> slice4/1, slice3/1, slice2/1, slice1/1
  slice4/1 -> reinterpret4/1
  reinterpret4/1 -> msb_out4/1
  slice3/1 -> reinterpret3/1
  reinterpret3/1 -> out3/1
  slice2/1 -> reinterpret2/1
  reinterpret2/1 -> out2/1
  slice1/1 -> reinterpret1/1
  reinterpret1/1 -> lsb_out1/1

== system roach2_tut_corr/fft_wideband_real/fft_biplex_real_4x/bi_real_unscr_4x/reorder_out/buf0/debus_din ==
  bus_in : Inport
  reinterpret{1..4} (4 alike) : xbsIndex_r4/Reinterpret  force_arith_type=on  arith_type=Unsigned  force_bin_pt=on  bin_pt=0  block_type=reinterpret
  slice1 : xbsIndex_r4/Slice  nbits=36  boolean_output=off  mode=Upper Bit Location + Width  bit1=-108  base1=MSB of Input  bit0=0  base0=LSB of Input  dbl_ovrd=off  block_type=slice
  slice2 : xbsIndex_r4/Slice  nbits=36  boolean_output=off  mode=Upper Bit Location + Width  bit1=-72  base1=MSB of Input  bit0=0  base0=LSB of Input  dbl_ovrd=off  block_type=slice
  slice3 : xbsIndex_r4/Slice  nbits=36  boolean_output=off  mode=Upper Bit Location + Width  bit1=-36  base1=MSB of Input  bit0=0  base0=LSB of Input  dbl_ovrd=off  block_type=slice
  slice4 : xbsIndex_r4/Slice  nbits=36  boolean_output=off  mode=Upper Bit Location + Width  bit1=0  base1=MSB of Input  bit0=0  base0=LSB of Input  dbl_ovrd=off  block_type=slice
  msb_out4 : Outport
  out3 : Outport  Port=2
  out2 : Outport  Port=3
  lsb_out1 : Outport  Port=4
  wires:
  bus_in/1 -> slice4/1, slice3/1, slice2/1, slice1/1
  slice4/1 -> reinterpret4/1
  reinterpret4/1 -> msb_out4/1
  slice3/1 -> reinterpret3/1
  reinterpret3/1 -> out3/1
  slice2/1 -> reinterpret2/1
  reinterpret2/1 -> out2/1
  slice1/1 -> reinterpret1/1
  reinterpret1/1 -> lsb_out1/1

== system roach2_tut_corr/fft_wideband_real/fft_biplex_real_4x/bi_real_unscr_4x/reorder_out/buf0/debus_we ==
  bus_in : Inport
  slice1 : xbsIndex_r4/Slice  nbits=1  boolean_output=on  mode=Upper Bit Location + Width  bit1=-3  base1=MSB of Input  bit0=0  base0=LSB of Input  dbl_ovrd=off  block_type=slice
  slice2 : xbsIndex_r4/Slice  nbits=1  boolean_output=on  mode=Upper Bit Location + Width  bit1=-2  base1=MSB of Input  bit0=0  base0=LSB of Input  dbl_ovrd=off  block_type=slice
  slice3 : xbsIndex_r4/Slice  nbits=1  boolean_output=on  mode=Upper Bit Location + Width  bit1=-1  base1=MSB of Input  bit0=0  base0=LSB of Input  dbl_ovrd=off  block_type=slice
  slice4 : xbsIndex_r4/Slice  nbits=1  boolean_output=on  mode=Upper Bit Location + Width  bit1=0  base1=MSB of Input  bit0=0  base0=LSB of Input  dbl_ovrd=off  block_type=slice
  msb_out4 : Outport
  out3 : Outport  Port=2
  out2 : Outport  Port=3
  lsb_out1 : Outport  Port=4
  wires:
  bus_in/1 -> slice4/1, slice3/1, slice2/1, slice1/1
  slice4/1 -> msb_out4/1
  slice3/1 -> out3/1
  slice2/1 -> out2/1
  slice1/1 -> lsb_out1/1

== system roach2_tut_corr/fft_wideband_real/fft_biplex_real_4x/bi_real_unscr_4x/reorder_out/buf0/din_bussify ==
  in1 : Inport
  in2 : Inport  Port=2
  in3 : Inport  Port=3
  in4 : Inport  Port=4
  concatenate : xbsIndex_r4/Concat  num_inputs=4  dbl_ovrd=off  block_type=concat
  reinterpret{1..4} (4 alike) : xbsIndex_r4/Reinterpret  force_arith_type=on  arith_type=Unsigned  force_bin_pt=on  bin_pt=0  block_type=reinterpret
  bus_out : Outport
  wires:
  concatenate/1 -> bus_out/1
  in1/1 -> reinterpret1/1
  reinterpret1/1 -> concatenate/1
  in2/1 -> reinterpret2/1
  reinterpret2/1 -> concatenate/2
  in3/1 -> reinterpret3/1
  reinterpret3/1 -> concatenate/3
  in4/1 -> reinterpret4/1
  reinterpret4/1 -> concatenate/4

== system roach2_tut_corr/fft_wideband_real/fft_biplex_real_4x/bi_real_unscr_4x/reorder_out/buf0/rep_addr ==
  in : Inport
  bussify : Subsystem  AncestorBlock=casper_library_flow_control/bus_create
  din0_0 : xbsIndex_r4/Delay  rst=off  infoeditControl=Selection of Reset will increase slice count due to use of real FFs and instead of SRLs  en=off  latency=1  dbl_ovrd=off  reg_retiming=off  block_type=delay
  din0_1 : xbsIndex_r4/Delay  rst=off  infoeditControl=Selection of Reset will increase slice count due to use of real FFs and instead of SRLs  en=off  latency=1  dbl_ovrd=off  reg_retiming=off  block_type=delay
  din1_{0..3} (4 alike) : xbsIndex_r4/Delay  rst=off  infoeditControl=Selection of Reset will increase slice count due to use of real FFs and instead of SRLs  en=off  latency=1  dbl_ovrd=off  reg_retiming=off  block_type=delay
  out : Outport
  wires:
  in/1 -> din0_0/1, din0_1/1
  din0_0/1 -> din1_0/1, din1_2/1
  din0_1/1 -> din1_1/1, din1_3/1
  din1_0/1 -> bussify/1(in1)
  din1_1/1 -> bussify/2(in2)
  din1_2/1 -> bussify/3(in3)
  din1_3/1 -> bussify/4(in4)
  bussify/1(bus_out) -> out/1

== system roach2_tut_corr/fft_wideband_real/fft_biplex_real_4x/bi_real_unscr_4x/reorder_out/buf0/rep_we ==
  in : Inport
  bussify : Subsystem  AncestorBlock=casper_library_flow_control/bus_create
  din0_0 : xbsIndex_r4/Delay  rst=off  infoeditControl=Selection of Reset will increase slice count due to use of real FFs and instead of SRLs  en=off  latency=1  dbl_ovrd=off  reg_retiming=off  block_type=delay
  din0_1 : xbsIndex_r4/Delay  rst=off  infoeditControl=Selection of Reset will increase slice count due to use of real FFs and instead of SRLs  en=off  latency=1  dbl_ovrd=off  reg_retiming=off  block_type=delay
  din1_{0..3} (4 alike) : xbsIndex_r4/Delay  rst=off  infoeditControl=Selection of Reset will increase slice count due to use of real FFs and instead of SRLs  en=off  latency=1  dbl_ovrd=off  reg_retiming=off  block_type=delay
  out : Outport
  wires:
  in/1 -> din0_0/1, din0_1/1
  din0_0/1 -> din1_0/1, din1_2/1
  din0_1/1 -> din1_1/1, din1_3/1
  din1_0/1 -> bussify/1(in1)
  din1_1/1 -> bussify/2(in2)
  din1_2/1 -> bussify/3(in3)
  din1_3/1 -> bussify/4(in4)
  bussify/1(bus_out) -> out/1

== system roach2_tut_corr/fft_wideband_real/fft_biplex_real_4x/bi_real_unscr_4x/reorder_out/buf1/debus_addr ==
  bus_in : Inport
  reinterpret{1..4} (4 alike) : xbsIndex_r4/Reinterpret  force_arith_type=on  arith_type=Unsigned  force_bin_pt=on  bin_pt=0  block_type=reinterpret
  slice1 : xbsIndex_r4/Slice  nbits=8  boolean_output=off  mode=Upper Bit Location + Width  bit1=-24  base1=MSB of Input  bit0=0  base0=LSB of Input  dbl_ovrd=off  block_type=slice
  slice2 : xbsIndex_r4/Slice  nbits=8  boolean_output=off  mode=Upper Bit Location + Width  bit1=-16  base1=MSB of Input  bit0=0  base0=LSB of Input  dbl_ovrd=off  block_type=slice
  slice3 : xbsIndex_r4/Slice  nbits=8  boolean_output=off  mode=Upper Bit Location + Width  bit1=-8  base1=MSB of Input  bit0=0  base0=LSB of Input  dbl_ovrd=off  block_type=slice
  slice4 : xbsIndex_r4/Slice  nbits=8  boolean_output=off  mode=Upper Bit Location + Width  bit1=0  base1=MSB of Input  bit0=0  base0=LSB of Input  dbl_ovrd=off  block_type=slice
  msb_out4 : Outport
  out3 : Outport  Port=2
  out2 : Outport  Port=3
  lsb_out1 : Outport  Port=4
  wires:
  bus_in/1 -> slice4/1, slice3/1, slice2/1, slice1/1
  slice4/1 -> reinterpret4/1
  reinterpret4/1 -> msb_out4/1
  slice3/1 -> reinterpret3/1
  reinterpret3/1 -> out3/1
  slice2/1 -> reinterpret2/1
  reinterpret2/1 -> out2/1
  slice1/1 -> reinterpret1/1
  reinterpret1/1 -> lsb_out1/1

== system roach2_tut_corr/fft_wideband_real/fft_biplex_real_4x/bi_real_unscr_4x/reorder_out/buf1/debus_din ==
  bus_in : Inport
  reinterpret{1..4} (4 alike) : xbsIndex_r4/Reinterpret  force_arith_type=on  arith_type=Unsigned  force_bin_pt=on  bin_pt=0  block_type=reinterpret
  slice1 : xbsIndex_r4/Slice  nbits=36  boolean_output=off  mode=Upper Bit Location + Width  bit1=-108  base1=MSB of Input  bit0=0  base0=LSB of Input  dbl_ovrd=off  block_type=slice
  slice2 : xbsIndex_r4/Slice  nbits=36  boolean_output=off  mode=Upper Bit Location + Width  bit1=-72  base1=MSB of Input  bit0=0  base0=LSB of Input  dbl_ovrd=off  block_type=slice
  slice3 : xbsIndex_r4/Slice  nbits=36  boolean_output=off  mode=Upper Bit Location + Width  bit1=-36  base1=MSB of Input  bit0=0  base0=LSB of Input  dbl_ovrd=off  block_type=slice
  slice4 : xbsIndex_r4/Slice  nbits=36  boolean_output=off  mode=Upper Bit Location + Width  bit1=0  base1=MSB of Input  bit0=0  base0=LSB of Input  dbl_ovrd=off  block_type=slice
  msb_out4 : Outport
  out3 : Outport  Port=2
  out2 : Outport  Port=3
  lsb_out1 : Outport  Port=4
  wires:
  bus_in/1 -> slice4/1, slice3/1, slice2/1, slice1/1
  slice4/1 -> reinterpret4/1
  reinterpret4/1 -> msb_out4/1
  slice3/1 -> reinterpret3/1
  reinterpret3/1 -> out3/1
  slice2/1 -> reinterpret2/1
  reinterpret2/1 -> out2/1
  slice1/1 -> reinterpret1/1
  reinterpret1/1 -> lsb_out1/1

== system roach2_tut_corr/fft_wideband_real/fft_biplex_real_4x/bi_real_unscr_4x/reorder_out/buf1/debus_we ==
  bus_in : Inport
  slice1 : xbsIndex_r4/Slice  nbits=1  boolean_output=on  mode=Upper Bit Location + Width  bit1=-3  base1=MSB of Input  bit0=0  base0=LSB of Input  dbl_ovrd=off  block_type=slice
  slice2 : xbsIndex_r4/Slice  nbits=1  boolean_output=on  mode=Upper Bit Location + Width  bit1=-2  base1=MSB of Input  bit0=0  base0=LSB of Input  dbl_ovrd=off  block_type=slice
  slice3 : xbsIndex_r4/Slice  nbits=1  boolean_output=on  mode=Upper Bit Location + Width  bit1=-1  base1=MSB of Input  bit0=0  base0=LSB of Input  dbl_ovrd=off  block_type=slice
  slice4 : xbsIndex_r4/Slice  nbits=1  boolean_output=on  mode=Upper Bit Location + Width  bit1=0  base1=MSB of Input  bit0=0  base0=LSB of Input  dbl_ovrd=off  block_type=slice
  msb_out4 : Outport
  out3 : Outport  Port=2
  out2 : Outport  Port=3
  lsb_out1 : Outport  Port=4
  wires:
  bus_in/1 -> slice4/1, slice3/1, slice2/1, slice1/1
  slice4/1 -> msb_out4/1
  slice3/1 -> out3/1
  slice2/1 -> out2/1
  slice1/1 -> lsb_out1/1

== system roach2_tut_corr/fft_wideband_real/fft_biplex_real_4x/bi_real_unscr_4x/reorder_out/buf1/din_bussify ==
  in1 : Inport
  in2 : Inport  Port=2
  in3 : Inport  Port=3
  in4 : Inport  Port=4
  concatenate : xbsIndex_r4/Concat  num_inputs=4  dbl_ovrd=off  block_type=concat
  reinterpret{1..4} (4 alike) : xbsIndex_r4/Reinterpret  force_arith_type=on  arith_type=Unsigned  force_bin_pt=on  bin_pt=0  block_type=reinterpret
  bus_out : Outport
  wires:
  concatenate/1 -> bus_out/1
  in1/1 -> reinterpret1/1
  reinterpret1/1 -> concatenate/1
  in2/1 -> reinterpret2/1
  reinterpret2/1 -> concatenate/2
  in3/1 -> reinterpret3/1
  reinterpret3/1 -> concatenate/3
  in4/1 -> reinterpret4/1
  reinterpret4/1 -> concatenate/4

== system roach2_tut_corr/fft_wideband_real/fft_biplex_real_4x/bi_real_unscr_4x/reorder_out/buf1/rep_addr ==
  in : Inport
  bussify : Subsystem  AncestorBlock=casper_library_flow_control/bus_create
  din0_0 : xbsIndex_r4/Delay  rst=off  infoeditControl=Selection of Reset will increase slice count due to use of real FFs and instead of SRLs  en=off  latency=1  dbl_ovrd=off  reg_retiming=off  block_type=delay
  din0_1 : xbsIndex_r4/Delay  rst=off  infoeditControl=Selection of Reset will increase slice count due to use of real FFs and instead of SRLs  en=off  latency=1  dbl_ovrd=off  reg_retiming=off  block_type=delay
  din1_{0..3} (4 alike) : xbsIndex_r4/Delay  rst=off  infoeditControl=Selection of Reset will increase slice count due to use of real FFs and instead of SRLs  en=off  latency=1  dbl_ovrd=off  reg_retiming=off  block_type=delay
  out : Outport
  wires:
  in/1 -> din0_0/1, din0_1/1
  din0_0/1 -> din1_0/1, din1_2/1
  din0_1/1 -> din1_1/1, din1_3/1
  din1_0/1 -> bussify/1(in1)
  din1_1/1 -> bussify/2(in2)
  din1_2/1 -> bussify/3(in3)
  din1_3/1 -> bussify/4(in4)
  bussify/1(bus_out) -> out/1

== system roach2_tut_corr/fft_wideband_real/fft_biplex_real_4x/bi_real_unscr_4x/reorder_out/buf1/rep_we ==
  in : Inport
  bussify : Subsystem  AncestorBlock=casper_library_flow_control/bus_create
  din0_0 : xbsIndex_r4/Delay  rst=off  infoeditControl=Selection of Reset will increase slice count due to use of real FFs and instead of SRLs  en=off  latency=1  dbl_ovrd=off  reg_retiming=off  block_type=delay
  din0_1 : xbsIndex_r4/Delay  rst=off  infoeditControl=Selection of Reset will increase slice count due to use of real FFs and instead of SRLs  en=off  latency=1  dbl_ovrd=off  reg_retiming=off  block_type=delay
  din1_{0..3} (4 alike) : xbsIndex_r4/Delay  rst=off  infoeditControl=Selection of Reset will increase slice count due to use of real FFs and instead of SRLs  en=off  latency=1  dbl_ovrd=off  reg_retiming=off  block_type=delay
  out : Outport
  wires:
  in/1 -> din0_0/1, din0_1/1
  din0_0/1 -> din1_0/1, din1_2/1
  din0_1/1 -> din1_1/1, din1_3/1
  din1_0/1 -> bussify/1(in1)
  din1_1/1 -> bussify/2(in2)
  din1_2/1 -> bussify/3(in3)
  din1_3/1 -> bussify/4(in4)
  bussify/1(bus_out) -> out/1
